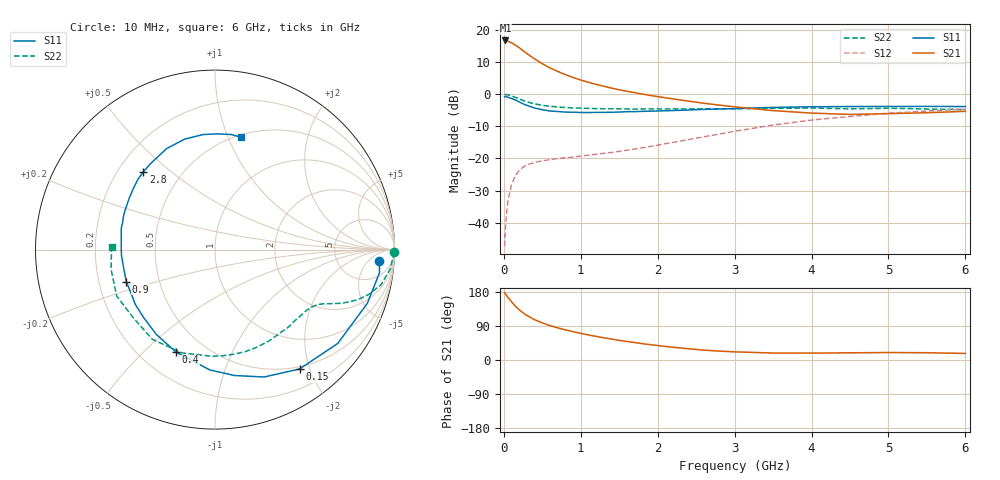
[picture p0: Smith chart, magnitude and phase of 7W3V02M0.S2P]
! Infineon Technologies  Discrete & RF Semiconductors
! BFS17W
! Si NPN RF Bipolar Junction Transistor in SOT323
! VCE = 3 V  IC = 2 mA
! Common Emitter S-Parameters:  August  1999
# GHz  S  MA  R  50
!  f  S11  S21  S12  S22
! GHz  MAG  ANG  MAG  ANG  MAG  ANG  MAG  ANG
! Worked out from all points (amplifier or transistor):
!   36 points, 10 MHz to 6 GHz, reference 50 ohm
!   highest |S21| = 16.8 dB at 20 MHz (marker M1)
!   |S21| within 3 dB of that: start of sweep to 239 MHz
!   unconditionally stable (mu >= 1): 816.2 MHz to end of sweep
!   at 250 MHz: K = 0.36, MSG = 18.1 dB, |S12| = -22.7 dB
!   at 1.4 GHz: K = 1.31, MAG = 6.7 dB, |S12| = -18.1 dB
!   at 6 GHz: K = 1.10, MAG = -2.3 dB, |S12| = -4.6 dB
!   S11 on the Smith chart (normalised r, x): 10 MHz: 15, -11; 150 MHz: 0.46, -1.84; 400 MHz: 0.35, -0.63; 900 MHz: 0.32, -0.16; 2.8 GHz: 0.30, +0.41; 6 GHz: 0.52, +1.12
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0.01  0.9182 -3.8  6.847 177.9  0.0043 88.9  0.9988 -0.8
0.02  0.9256 -8.0  6.891 174.6  0.0083 86.6  0.9926 -2.6
0.05  0.9001 -19.4  6.728 166.1  0.0208 79.4  0.9823 -6.3
0.1  0.8609 -37.4  6.334 153.7  0.0392 69.6  0.946 -11.9
0.15  0.815 -54.7  5.836 142.0  0.0535 61.0  0.8947 -16.1
0.2  0.7608 -68.9  5.309 132.5  0.0653 55.2  0.8452 -19.2
0.25  0.7099 -81.2  4.763 124.4  0.073 49.9  0.7999 -21.4
0.3  0.671 -92.5  4.302 117.5  0.0795 46.6  0.7646 -23.0
0.4  0.6111 -110.8  3.552 106.3  0.0869 41.9  0.7082 -25.2
0.5  0.5746 -124.7  2.993 97.9  0.0919 39.6  0.6738 -26.6
0.6  0.5493 -136.2  2.576 90.8  0.0958 39.0  0.65 -28.1
0.7  0.5387 -145.5  2.267 84.8  0.0997 39.1  0.6336 -29.8
0.9  0.5255 -160.2  1.825 74.8  0.1051 40.7  0.612 -33.5
1.1  0.5192 -171.7  1.535 66.0  0.1129 43.8  0.602 -37.9
1.4  0.5244 174.9  1.247 55.2  0.1238 48.6  0.5951 -45.1
1.6  0.5356 167.1  1.11 48.8  0.1344 52.0  0.5898 -50.5
2.2  0.5579 148.7  0.847 33.6  0.1782 60.1  0.592 -67.6
2.8  0.5897 132.5  0.678 23.5  0.2401 62.5  0.5932 -86.0
3.5  0.624 115.6  0.556 18.4  0.3314 59.3  0.604 -107.7
4.5  0.6445 95.9  0.485 19.0  0.4503 47.6  0.5932 -140.7
5.5  0.6475 82.1  0.516 19.2  0.5485 34.9  0.5893 -169.2
6  0.6435 76.9  0.542 17.3  0.586 28.9  0.5766 178.3
